(* Logix 5000 AddOnInstructionDefinition export BMC_AOI_PROC_BNI_XGx_x067_S5KV33_0325US; software revision 20.05 *)

TYPE BMC_UDT_BNI_XGx_x067_S5KV33_0325US :
STRUCT
   I : BMC_UDT_BNI_XGx_x067_IN_0325US;   // Master Input Data
   O : BMC_UDT_BNI_XGx_x067_OUT_0325US;   // Master Output Data
   C : BMC_UDT_BNI_XGx_x067_Config_0325US;   // Master Configuration Data
END_STRUCT
END_TYPE

TYPE BMC_UDT_BNI_XGx_x067_Dispaly_0325US :
STRUCT
   Red : BOOL;   // Set Display LEDs to Red
   Green : BOOL;   // Set Display LEDs to Green
   Lock : BOOL;   // Set Display Lock
END_STRUCT
END_TYPE

TYPE BMC_UDT_BNI_XGx_x067_OUT_0325US :
STRUCT
   DO : BMC_UDT_BNI_XGx_x067_Port_Pin_0325US;   // Master Digital Output
   Restart : BMC_UDT_BNI_XGx_x067_Port_Pin_0325US;   // Overload Restart
   Display : BMC_UDT_BNI_XGx_x067_Dispaly_0325US;   // Display LED and Display Lock
END_STRUCT
END_TYPE

TYPE BMC_UDT_BNI_XGx_x067_PortIOLDIag_0325US :
STRUCT
   X01 : BMC_UDT_BNI_XGx_x067_IOLDiagSub_0325US;   // IO-Link Diagnostics Port X01
   X02 : BMC_UDT_BNI_XGx_x067_IOLDiagSub_0325US;   // IO-Link Diagnostics Port X02
   X03 : BMC_UDT_BNI_XGx_x067_IOLDiagSub_0325US;   // IO-Link Diagnostics Port X03
   X04 : BMC_UDT_BNI_XGx_x067_IOLDiagSub_0325US;   // IO-Link Diagnostics Port X04
   X05 : BMC_UDT_BNI_XGx_x067_IOLDiagSub_0325US;   // IO-Link Diagnostics Port X05
   X06 : BMC_UDT_BNI_XGx_x067_IOLDiagSub_0325US;   // IO-Link Diagnostics Port X06
   X07 : BMC_UDT_BNI_XGx_x067_IOLDiagSub_0325US;   // IO-Link Diagnostics Port X07
   X08 : BMC_UDT_BNI_XGx_x067_IOLDiagSub_0325US;   // IO-Link Diagnostics Port X08
END_STRUCT
END_TYPE

TYPE BMC_UDT_BNI_XGx_x067_IOLDiagSub_0325US :
STRUCT
   Port_in_IOL_Mode : BOOL;   // Port in IO-Link Mode
   Device_Connected : BOOL;   // IO-Link Device Connected to Port
   Reserved_02 : BOOL;   // Reserved
   Reserved_03 : BOOL;   // Reserved
   Reserved_04 : BOOL;   // Reserved
   Reserved_05 : BOOL;   // Reserved
   Reserved_06 : BOOL;   // Reserved
   Reserved_07 : BOOL;   // Reserved
   Validation_Failed : BOOL;   // Validation Failed - Vendor or Device ID does not match conencted device
   DS_Validation_Failed : BOOL;   // Parameter Server Failed
   Process_Data_Invalid : BOOL;   // IO-Link Device Process Data Invalid
   Reserved_11 : BOOL;   // Reserved
   Reserved_12 : BOOL;   // Reserved
   Reserved_13 : BOOL;   // Reserved
   Reserved_14 : BOOL;   // Reserved
   IOL_Short_Circuit : BOOL;   // Short between Pin 4 and Pin 3 when in IO-Link Mode
   Vendor_ID_1 : SINT;   // Vendor ID
   Vendor_ID_2 : SINT;   // Vendor ID
   Device_ID_1 : SINT;   // Device ID
   Device_ID_2 : SINT;   // Device ID
   Device_ID_3 : SINT;   // Device ID
   Event_1_Mode_Type : SINT;   // Event Mode and Type
   Event_1_Code_High : SINT;   // Event Code High Byte
   Event_1_Code_Low : SINT;   // Event Code Low Byte
   Event_2_Mode_Type : SINT;   // Event Mode and Type
   Event_2_Code_High : SINT;   // Event Code High Byte
   Event_2_Code_Low : SINT;   // Event Code Low Byte
   Event_3_Mode_Type : SINT;   // Event Mode and Type
   Event_3_Code_High : SINT;   // Event Code High Byte
   Event_3_Code_Low : SINT;   // Event Code Low Byte
END_STRUCT
END_TYPE

TYPE BMC_UDT_BNI_XGx_x067_Config_0325US :
STRUCT
   Port_X01_Pin_4_Mode : BOOL;   // 0 - Disable IO-Link 1- Enable IO-Link
   Port_X01_Pin_2_Mode : BOOL;   // 0 - Pin 2 is switchable 1 - Pin 2 is ON Constant
   Port_X02_Pin_4_Mode : BOOL;   // 0 - Disable IO-Link 1- Enable IO-Link
   Port_X02_Pin_2_Mode : BOOL;   // 0 - Pin 2 is switchable 1 - Pin 2 is ON Constant
   Port_X03_Pin_4_Mode : BOOL;   // 0 - Disable IO-Link 1- Enable IO-Link
   Port_X03_Pin_2_Mode : BOOL;   // 0 - Pin 2 is switchable 1 - Pin 2 is ON Constant
   Port_X04_Pin_4_Mode : BOOL;   // 0 - Disable IO-Link 1- Enable IO-Link
   Port_X04_Pin_2_Mode : BOOL;   // 0 - Pin 2 is switchable 1 - Pin 2 is ON Constant
   Port_X05_Pin_4_Mode : BOOL;   // 0 - Disable IO-Link 1- Enable IO-Link
   Port_X05_Pin_2_Mode : BOOL;   // 0 - Pin 2 is switchable 1 - Pin 2 is ON Constant
   Port_X06_Pin_4_Mode : BOOL;   // 0 - Disable IO-Link 1- Enable IO-Link
   Port_X06_Pin_2_Mode : BOOL;   // 0 - Pin 2 is switchable 1 - Pin 2 is ON Constant
   Port_X07_Pin_4_Mode : BOOL;   // 0 - Disable IO-Link 1- Enable IO-Link
   Port_X07_Pin_2_Mode : BOOL;   // 0 - Pin 2 is switchable 1 - Pin 2 is ON Constant
   Port_X08_Pin_4_Mode : BOOL;   // 0 - Disable IO-Link 1- Enable IO-Link
   Port_X08_Pin_2_Mode : BOOL;   // 0 - Pin 2 is switchable 1 - Pin 2 is ON Constant
   Port_X01_Cycle_Time : SINT;   // Set Cycle Time (0 = Fastest Update Rate)
   Port_X01_Validation_Backup : SINT;   // 0 - No Validation or Parameter Server 1 - Validation Device 1.0 2 - Validation Device 1.1 3 - Parameter Server - Backup and Restore 4 - Parameter Server - Restore
   Port_X01_Vendor_ID_1 : SINT;   // Vendor ID High Byte - Used with Validation and Backup Parameter
   Port_X01_Vendor_ID_2 : SINT;   // Vendor ID Low Byte - Used with Validation and Backup Parameter
   Port_X01_Device_ID_1 : SINT;   // Device ID High Byte - Used with Validation and Backup Parameter
   Port_X01_Device_ID_2 : SINT;   // Device ID Middle Byte - Used with Validation and Backup Parameter
   Port_X01_Device_ID_3 : SINT;   // Device ID Low Byte - Used with Validation and Backup Parameter
   Port_X02_Cycle_Time : SINT;   // Set Cycle Time (0 = Fastest Update Rate)
   Port_X02_Validation_Backup : SINT;   // 0 - No Validation or Parameter Server 1 - Validation Device 1.0 2 - Validation Device 1.1 3 - Parameter Server - Backup and Restore 4 - Parameter Server - Restore
   Port_X02_Vendor_ID_1 : SINT;   // Vendor ID High Byte - Used with Validation and Backup Parameter
   Port_X02_Vendor_ID_2 : SINT;   // Vendor ID Low Byte - Used with Validation and Backup Parameter
   Port_X02_Device_ID_1 : SINT;   // Device ID High Byte - Used with Validation and Backup Parameter
   Port_X02_Device_ID_2 : SINT;   // Device ID Middle Byte - Used with Validation and Backup Parameter
   Port_X02_Device_ID_3 : SINT;   // Device ID Low Byte - Used with Validation and Backup Parameter
   Port_X03_Cycle_Time : SINT;   // Set Cycle Time (0 = Fastest Update Rate)
   Port_X03_Validation_Backup : SINT;   // 0 - No Validation or Parameter Server 1 - Validation Device 1.0 2 - Validation Device 1.1 3 - Parameter Server - Backup and Restore 4 - Parameter Server - Restore
   Port_X03_Vendor_ID_1 : SINT;   // Vendor ID High Byte - Used with Validation and Backup Parameter
   Port_X03_Vendor_ID_2 : SINT;   // Vendor ID Low Byte - Used with Validation and Backup Parameter
   Port_X03_Device_ID_1 : SINT;   // Device ID High Byte - Used with Validation and Backup Parameter
   Port_X03_Device_ID_2 : SINT;   // Device ID Middle Byte - Used with Validation and Backup Parameter
   Port_X03_Device_ID_3 : SINT;   // Device ID Low Byte - Used with Validation and Backup Parameter
   Port_X04_Cycle_Time : SINT;   // Set Cycle Time (0 = Fastest Update Rate)
   Port_X04_Validation_Backup : SINT;   // 0 - No Validation or Parameter Server 1 - Validation Device 1.0 2 - Validation Device 1.1 3 - Parameter Server - Backup and Restore 4 - Parameter Server - Restore
   Port_X04_Vendor_ID_1 : SINT;   // Vendor ID High Byte - Used with Validation and Backup Parameter
   Port_X04_Vendor_ID_2 : SINT;   // Vendor ID Low Byte - Used with Validation and Backup Parameter
   Port_X04_Device_ID_1 : SINT;   // Device ID High Byte - Used with Validation and Backup Parameter
   Port_X04_Device_ID_2 : SINT;   // Device ID Middle Byte - Used with Validation and Backup Parameter
   Port_X04_Device_ID_3 : SINT;   // Device ID Low Byte - Used with Validation and Backup Parameter
   Port_X05_Cycle_Time : SINT;   // Set Cycle Time (0 = Fastest Update Rate)
   Port_X05_Validation_Backup : SINT;   // 0 - No Validation or Parameter Server 1 - Validation Device 1.0 2 - Validation Device 1.1 3 - Parameter Server - Backup and Restore 4 - Parameter Server - Restore
   Port_X05_Vendor_ID_1 : SINT;   // Vendor ID High Byte - Used with Validation and Backup Parameter
   Port_X05_Vendor_ID_2 : SINT;   // Vendor ID Low Byte - Used with Validation and Backup Parameter
   Port_X05_Device_ID_1 : SINT;   // Device ID High Byte - Used with Validation and Backup Parameter
   Port_X05_Device_ID_2 : SINT;   // Device ID Middle Byte - Used with Validation and Backup Parameter
   Port_X05_Device_ID_3 : SINT;   // Device ID Low Byte - Used with Validation and Backup Parameter
   Port_X06_Cycle_Time : SINT;   // Set Cycle Time (0 = Fastest Update Rate)
   Port_X06_Validation_Backup : SINT;   // 0 - No Validation or Parameter Server 1 - Validation Device 1.0 2 - Validation Device 1.1 3 - Parameter Server - Backup and Restore 4 - Parameter Server - Restore
   Port_X06_Vendor_ID_1 : SINT;   // Vendor ID High Byte - Used with Validation and Backup Parameter
   Port_X06_Vendor_ID_2 : SINT;   // Vendor ID Low Byte - Used with Validation and Backup Parameter
   Port_X06_Device_ID_1 : SINT;   // Device ID High Byte - Used with Validation and Backup Parameter
   Port_X06_Device_ID_2 : SINT;   // Device ID Middle Byte - Used with Validation and Backup Parameter
   Port_X06_Device_ID_3 : SINT;   // Device ID Low Byte - Used with Validation and Backup Parameter
   Port_X07_Cycle_Time : SINT;   // Set Cycle Time (0 = Fastest Update Rate)
   Port_X07_Validation_Backup : SINT;   // 0 - No Validation or Parameter Server 1 - Validation Device 1.0 2 - Validation Device 1.1 3 - Parameter Server - Backup and Restore 4 - Parameter Server - Restore
   Port_X07_Vendor_ID_1 : SINT;   // Vendor ID High Byte - Used with Validation and Backup Parameter
   Port_X07_Vendor_ID_2 : SINT;   // Vendor ID Low Byte - Used with Validation and Backup Parameter
   Port_X07_Device_ID_1 : SINT;   // Device ID High Byte - Used with Validation and Backup Parameter
   Port_X07_Device_ID_2 : SINT;   // Device ID Middle Byte - Used with Validation and Backup Parameter
   Port_X07_Device_ID_3 : SINT;   // Device ID Low Byte - Used with Validation and Backup Parameter
   Port_X08_Cycle_Time : SINT;   // Set Cycle Time (0 = Fastest Update Rate)
   Port_X08_Validation_Backup : SINT;   // 0 - No Validation or Parameter Server 1 - Validation Device 1.0 2 - Validation Device 1.1 3 - Parameter Server - Backup and Restore 4 - Parameter Server - Restore
   Port_X08_Vendor_ID_1 : SINT;   // Vendor ID High Byte - Used with Validation and Backup Parameter
   Port_X08_Vendor_ID_2 : SINT;   // Vendor ID Low Byte - Used with Validation and Backup Parameter
   Port_X08_Device_ID_1 : SINT;   // Device ID High Byte - Used with Validation and Backup Parameter
   Port_X08_Device_ID_2 : SINT;   // Device ID Middle Byte - Used with Validation and Backup Parameter
   Port_X08_Device_ID_3 : SINT;   // Device ID Low Byte - Used with Validation and Backup Parameter
END_STRUCT
END_TYPE

TYPE BMC_UDT_BNI_XGx_x067_Power_0325US :
STRUCT
   UA_Low : BOOL;   // UA Power Low (Less than 18 Volts)
   US_Low : BOOL;   // US Power Low (Less than 18 Volts)
   No_UA : BOOL;   // No UA Power (Less than 11 Volts)
END_STRUCT
END_TYPE

TYPE IO_Link_Port_Data :
STRUCT
   Inputs : SINT[48];
   Outputs : SINT[48];
END_STRUCT
END_TYPE

TYPE BMC_UDT_BNI_XGx_x067_Port_Pin_0325US :
STRUCT
   X01_00 : BOOL;   // Port X01 LED 00 (Pin 4)
   X01_01 : BOOL;   // Port X01 LED 01 (Pin 2)
   X02_00 : BOOL;   // Port X02 LED 00 (Pin 4)
   X02_01 : BOOL;   // Port X02 LED 01 (Pin 2)
   X03_00 : BOOL;   // Port X03 LED 00 (Pin 4)
   X03_01 : BOOL;   // Port X03 LED 01 (Pin 2)
   X04_00 : BOOL;   // Port X04 LED 00 (Pin 4)
   X04_01 : BOOL;   // Port X04 LED 01 (Pin 2)
   X05_00 : BOOL;   // Port X05 LED 00 (Pin 4)
   X05_01 : BOOL;   // Port X05 LED 01 (Pin 2)
   X06_00 : BOOL;   // Port X06 LED 00 (Pin 4)
   X06_01 : BOOL;   // Port X06 LED 01 (Pin 2)
   X07_00 : BOOL;   // Port X07 LED 00 (Pin 4)
   X07_01 : BOOL;   // Port X07 LED 01 (Pin 2)
   X08_00 : BOOL;   // Port X08 LED 00 (Pin 4)
   X08_01 : BOOL;   // Port X08 LED 01 (Pin 2)
END_STRUCT
END_TYPE

TYPE BMC_UDT_BNI_XGx_x067_IN_0325US :
STRUCT
   DI : BMC_UDT_BNI_XGx_x067_Port_Pin_0325US;   // Master Digital Inputs
   Short_Circuit : BMC_UDT_BNI_XGx_x067_Port_Pin_0325US;   // Master Short Circuit Diagnostic
   Overload : BMC_UDT_BNI_XGx_x067_Port_Pin_0325US;   // Master Overload Diagnostic
   Power_Fault : BMC_UDT_BNI_XGx_x067_Power_0325US;   // Master Power Diagnostic
   IOL_Diag : BMC_UDT_BNI_XGx_x067_PortIOLDIag_0325US;   // IO-Link Port Diagnostic
END_STRUCT
END_TYPE

ADD_ON_INSTRUCTION BMC_AOI_PROC_BNI_XGx_x067_S5KV33_0325US   (* revision 4.0 0325US, vendor Balluff Inc *)
// BNI XGx-5xx-xxx-x067 AOI for use with RSlogix version 18-20 and Studio 5K Version 34 and 35 if version 36 is not installed on user's PC.
// Revision note:
// -3.0 Release for testing
// -4.0 Initial Release
VAR_IN_OUT
   BNI_XGx_x067_Raw_Input_Data : SINT[392]; {required}
        [0].0   // Input Port 0 Pin 4
        [0].1   // Input Port 0 Pin 2
        [0].2   // Input Port 1 Pin 4
        [0].3   // Input Port 1 Pin 2
        [0].4   // Input Port 2 Pin 4
        [0].5   // Input Port 2 Pin 2
        [0].6   // Input Port 3 Pin 4
        [0].7   // Input Port 3 Pin 2
        [1].0   // Input Port 4 Pin 4
        [1].1   // Input Port 4 Pin 2
        [1].2   // Input Port 5 Pin 4
        [1].3   // Input Port 5 Pin 2
        [1].4   // Input Port 6 Pin 4
        [1].5   // Input Port 6 Pin 2
        [1].6   // Input Port 7 Pin 4
        [1].7   // Input Port 7 Pin 2
        [2].0   // Port 0 Pin 4 Short Circuit
        [2].1   // Port 0 Pin 2 Short Circuit
        [2].2   // Port 1 Pin 4 Short Circuit
        [2].3   // Port 1 Pin 2 Short Circuit
        [2].4   // Port 2 Pin 4 Short Circuit
        [2].5   // Port 2 Pin 2 Short Circuit
        [2].6   // Port 3 Pin 4 Short Circuit
        [2].7   // Port 3 Pin 2 Short Circuit
        [3].0   // Port 4 Pin 4 Short Circuit
        [3].1   // Port 4 Pin 2 Short Circuit
        [3].2   // Port 5 Pin 4 Short Circuit
        [3].3   // Port 5 Pin 2 Short Circuit
        [3].4   // Port 6 Pin 4 Short Circuit
        [3].5   // Port 6 Pin 2 Short Circuit
        [3].6   // Port 7 Pin 4 Short Circuit
        [3].7   // Port 7 Pin 2 Short Circuit
        [4].0   // Port 0 Pin 4 Output Overload Status
        [4].1   // Port 0 Pin 2 Output Overload Status
        [4].2   // Port 1 Pin 4 Output Overload Status
        [4].3   // Port 1 Pin 2 Output Overload Status
        [4].4   // Port 2 Pin 4 Output Overload Status
        [4].5   // Port 2 Pin 2 Output Overload Status
        [4].6   // Port 3 Pin 4 Output Overload Status
        [4].7   // Port 3 Pin 2 Output Overload Status
        [5].0   // Port 4 Pin 4 Output Overload Status
        [5].1   // Port 4 Pin 2 Output Overload Status
        [5].2   // Port 5 Pin 4 Output Overload Status
        [5].3   // Port 5 Pin 2 Output Overload Status
        [5].4   // Port 6 Pin 4 Output Overload Status
        [5].5   // Port 6 Pin 2 Output Overload Status
        [5].6   // Port 7 Pin 4 Output Overload Status
        [5].7   // Port 7 Pin 2 Output Overload Status
        [6].0   // Output Power from Aux Power cable Under Voltage
        [6].1   // Module Power from IO-Link Communication Cable Under Voltage
        [6].2   // Not used
        [6].3   // Not used
        [6].4   // Not used
        [6].5   // Not used
        [6].6   // Not used
        [6].7   // Not used
        [7]   // Port 1 Input Byte 0
        [8]   // Port 1 Input Byte 1
        [9]   // Port 1 Input Byte 2
        [10]   // Port 1 Input Byte 3
        [11]   // Port 1 Input Byte 4
        [32].0   // Port 1 EP bit Event Present
        [32].1   // Reserved
        [32].2   // Reserved
        [32].3   // Reserved
        [32].4   // Reserved
        [32].5   // Port 1 VF bit Validation Failed
        [32].6   // Port 1 DC bit Device Connected
        [32].7   // Port 1 IOL bit Port in IO-Link Mode
        [33].0   // Reserved
        [33].1   // Reserved
        [33].2   // Reserved
        [33].3   // Reserved
        [33].4   // Reserved
        [33].5   // Reserved
        [33].6   // Reserved
        [33].7   // Reserved
        [34]   // Port 1 Vendor ID Number Byte 1 (High byte)
        [35]   // Port 1 Vendor ID Number Byte 2 (Middle byte)
        [36]   // Port 1 Vendor ID Number Byte 3 (Low byte)
        [37]   // Port 1 Device ID Number Byte 1 (High byte)
        [38]   // Port 1 Device ID Number Byte 2 (Middle byte)
        [39]   // Port 1 Device ID Number Byte 3 (Low byte)
        [40].0   // Port 1 In I/O Link Mode
        [40].1   // Port 1 I/O Link Device Connected
        [41].0   // Port 1 I/O Link Device Configuration Mismatch
        [52]   // Port 1 Input Byte 46
        [53]   // Port 1 Input Byte 47
        [54]   // Port 1 Input Byte 48
        [55]   // Port 2 Input Byte 0
        [56]   // Port 2 Input Byte 1
        [57]   // Port 2 Input Byte 2
        [58]   // Port 2 Input Byte 3
        [59]   // Port 2 Input Byte 4
        [88].0   // Port 2 In I/O Link Mode
        [88].1   // Port 2 I/O Link Device Connected
        [89].0   // Port 2 I/O Link Device Configuration Mismatch
        [100]   // Port 2 Input Byte 46
        [101]   // Port 2 Input Byte 47
        [102]   // Port 2 Input Byte 48
        [103]   // Port 3 Input Byte 0
        [104]   // Port 3 Input Byte 1
        [105]   // Port 3 Input Byte 2
        [106]   // Port 3 Input Byte 3
        [107]   // Port 3 Input Byte 4
        [136].0   // Port 3 In I/O Link Mode
        [136].1   // Port 3 I/O Link Device Connected
        [137].0   // Port 3 I/O Link Device Configuration Mismatch
        [148]   // Port 3 Input Byte 46
        [149]   // Port 3 Input Byte 47
        [150]   // Port 3 Input Byte 48
        [151]   // Port 4 Input Byte 0
        [152]   // Port 4 Input Byte 1
        [153]   // Port 4 Input Byte 2
        [154]   // Port 4 Input Byte 3
        [184].0   // Port 4 In I/O Link Mode
        [184].1   // Port 4 I/O Link Device Connected
        [185].0   // Port 4 I/O Link Device Configuration Mismatch
        [196]   // Port 4 Input Byte 46
        [197]   // Port 4 Input Byte 47
        [198]   // Port 4 Input Byte 48
   BNI_XGx_x067_Raw_Output_Data : SINT[262]; {required}
        [0].0   // Output Port 0 Pin 4
        [0].1   // Output Port 0 Pin 2
        [0].2   // Output Port 1 Pin 4
        [0].3   // Output Port 1 Pin 2
        [0].4   // Output Port 2 Pin 4
        [0].5   // Output Port 2 Pin 2
        [0].6   // Output Port 3 Pin 4
        [0].7   // Output Port 3 Pin 2
        [1].0   // Output Port 4 Pin 4
        [1].1   // Output Port 4 Pin 2
        [1].2   // Output Port 5 Pin 4
        [1].3   // Output Port 5 Pin 2
        [1].4   // Output Port 6 Pin 4
        [1].5   // Output Port 6 Pin 2
        [1].6   // Output Port 7 Pin 4
        [1].7   // Output Port 7 Pin 2
        [2].0   // Port 0 Pin 4 Output Restart
        [2].1   // Port 0 Pin 2 Output Restart
        [2].2   // Port 1 Pin 4 Output Restart
        [2].3   // Port 1 Pin 2 Output Restart
        [2].4   // Port 2 Pin 4 Output Restart
        [2].5   // Port 2 Pin 2 Output Restart
        [2].6   // Port 3 Pin 4 Output Restart
        [2].7   // Port 3 Pin 2 Output Restart
        [3].0   // Port 4 Pin 4 Output Restart
        [3].1   // Port 4 Pin 2 Output Restart
        [3].2   // Port 5 Pin 4 Output Restart
        [3].3   // Port 5 Pin 2 Output Restart
        [3].4   // Port 6 Pin 4 Output Restart
        [3].5   // Port 6 Pin 2 Output Restart
        [3].6   // Port 7 Pin 4 Output Restart
        [3].7   // Port 7 Pin 2 Output Restart
        [4].0   // Red LED Display Output
        [4].1   // Green LED Display Output
        [4].2   // Lock Display Output
        [5]   // Port 1 Output Data Byte 0
        [6]   // Port 1 Output Data Byte 1
        [7]   // Port 1 Output Data Byte 2
        [8]   // Port 1 Output Data Byte 3
        [9]   // Port 1 Output Data Byte 4
        [10]   // Port 1 Output Data Byte 5
        [11]   // Port 1 Output Data Byte 6
        [12]   // Port 1 Output Data Byte 7
        [13]   // Port 1 Output Data Byte 8
        [14]   // Port 1 Output Data Byte 9
        [15]   // Port 1 Output Data Byte 10
        [16]   // Port 1 Output Data Byte 11
        [17]   // Port 1 Output Data Byte 12
        [18]   // Port 1 Output Data Byte 13
        [19]   // Port 1 Output Data Byte 14
        [20]   // Port 1 Output Data Byte 15
        [21]   // Port 1 Output Data Byte 16
        [22]   // Port 1 Output Data Byte 17
        [23]   // Port 1 Output Data Byte 18
        [24]   // Port 1 Output Data Byte 19
        [25]   // Port 1 Output Data Byte 20
        [26]   // Port 1 Output Data Byte 21
        [27]   // Port 1 Output Data Byte 22
        [28]   // Port 1 Output Data Byte 23
        [29]   // Port 1 Output Data Byte 24
        [30]   // Port 1 Output Data Byte 25
        [31]   // Port 1 Output Data Byte 26
        [32]   // Port 1 Output Data Byte 27
        [33]   // Port 1 Output Data Byte 28
        [34]   // Port 1 Output Data Byte 29
        [35]   // Port 1 Output Data Byte 30
        [36]   // Port 1 Output Data Byte 31
        [37]   // Port 2 Output Data Byte 0
        [38]   // Port 2 Output Data Byte 1
        [69]   // Port 3 Output Data Byte 0
        [70]   // Port 3 Output Data Byte 1
        [101]   // Port 4 Output Data Byte 0
        [102]   // Port 4 Output Data Byte 1
   BNI_XGx_x067_Raw_Config_Data : SINT[58]; {required}
        [1]   // Port 5 (Bits 0_1) Port 6 (Bits 2_3) Port 7 (Bits 4_5) Port 8 (Bits 6_7) Function Function 00d=0x00=Standrd I/O 01d=0x01=IO-Link Mod 02d=0x02=Fallback Md
        [2].0   // Parameter Data Conflict
        [2].1   // Enable Parameter Upload
        [2].2   // Enable Parameter Download
        [2].7   // Enable Parameter Server
        [3]   // RESERVED
        [4]   // Port 1 IO-Link Cycle Time Time (Bytes 5-0) Base (Bytes 7-6)
        [5]   // Port 1 Vendor ID Number Byte 1 High Byte
        [6]   // Port 1 Vendor ID Number Byte 2 Low Byte
        [7]   // Port 1 Device ID Number Byte 1 High Byte
        [8]   // Port 1 Device ID Number Byte 2 Middle Byte
        [9]   // Port 1 Device ID Number Byte 3 Low Byte
        [10]   // Port 2 IO-Link Cycle Time Time (Bytes 5-0) Base (Bytes 7-6)
        [11]   // Port 2 Vendor ID Number Byte 1 High Byte
        [12]   // Port 2 Vendor ID Number Byte 2 Low Byte
        [13]   // Port 2 Device ID Number Byte 1 High Byte
        [14]   // Port 2 Device ID Number Byte 2 Middle Byte
        [15]   // Port 2 Device ID Number Byte 3 Low Byte
        [16]   // Port 3 IO-Link Cycle Time Time (Bytes 5-0) Base (Bytes 7-6)
        [17]   // Port 3 Vendor ID Number Byte 1 High Byte
        [18]   // Port 3 Vendor ID Number Byte 2 Low Byte
        [19]   // Port 3 Device ID Number Byte 1 High Byte
        [20]   // Port 3 Device ID Number Byte 2 Middle Byte
        [21]   // Port 3 Device ID Number Byte 3 Low Byte
        [22]   // Port 4 IO-Link Cycle Time Time (Bytes 5-0) Base (Bytes 7-6)
        [23]   // Port 4 Vendor ID Number Byte 1 High Byte
        [24]   // Port 4 Vendor ID Number Byte 2 Low Byte
        [25]   // Port 1 Enable
        [25].1   // Port 1 Enable Upload Parameters
        [25].2   // Port 1 Enable Download Parameters
        [25].7   // Port 1 Enable Parameters Server
        [26]   // Port 4 Device ID Number Byte 2 Middle Byte
        [27]   // Port 4 Device ID Number Byte 3 Low Byte
        [49].1   // Port 2 Enable Upload Parameters
        [49].2   // Port 2 Enable Download Parameters
        [49].7   // Port 2 Enable Parameters Server
   BNI_XGx_x067_Port_X01_Data : IO_Link_Port_Data; {required}
        .INPUTS[0]   // Port X01 Input Data
   BNI_XGx_x067_Port_X02_Data : IO_Link_Port_Data; {required}
        .INPUTS[0]   // Port X02 Input Data
   BNI_XGx_x067_Port_X03_Data : IO_Link_Port_Data; {required}
        .INPUTS[0]   // Port X03 Input Data
   BNI_XGx_x067_Port_X04_Data : IO_Link_Port_Data; {required}
        .INPUTS[0]   // Port X04 Input Data
   BNI_XGx_x067_Port_X05_Data : IO_Link_Port_Data; {required}
   BNI_XGx_x067_Port_X06_Data : IO_Link_Port_Data; {required}
   BNI_XGx_x067_Port_X07_Data : IO_Link_Port_Data; {required}
   BNI_XGx_x067_Port_X08_Data : IO_Link_Port_Data; {required}
   Mapped_BNI_XGx_R067_Data : BMC_UDT_BNI_XGx_x067_S5KV33_0325US; {required}
END_VAR

ROUTINE Logic   (* ladder *)
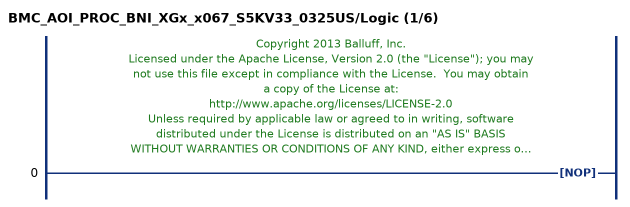
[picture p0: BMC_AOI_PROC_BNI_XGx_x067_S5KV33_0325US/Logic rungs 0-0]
   // Copyright 2013 Balluff, Inc.
   // Licensed under the Apache License, Version 2.0 (the "License"); you may
   // not use this file except in compliance with the License.  You may obtain
   // a copy of the License at:
   // http://www.apache.org/licenses/LICENSE-2.0
   // Unless required by applicable law or agreed to in writing, software
   // distributed under the License is distributed on an "AS IS" BASIS
   // WITHOUT WARRANTIES OR CONDITIONS OF ANY KIND, either express or
   // implied.  See the License for the specific language governing
   // permissions and limitations under the License.
   0: NOP();
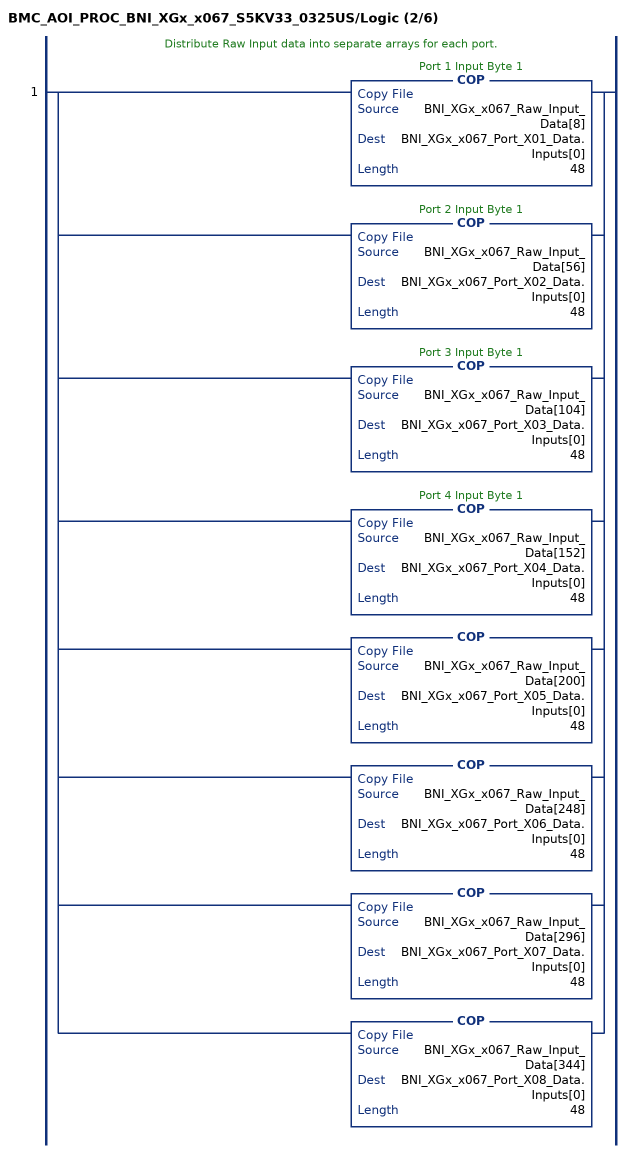
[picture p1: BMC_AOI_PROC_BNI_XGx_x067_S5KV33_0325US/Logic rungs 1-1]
   // Distribute Raw Input data into separate arrays for each port.
   1: [COP(BNI_XGx_x067_Raw_Input_Data[8],BNI_XGx_x067_Port_X01_Data.Inputs[0],48) ,COP(BNI_XGx_x067_Raw_Input_Data[56],BNI_XGx_x067_Port_X02_Data.Inputs[0],48) ,COP(BNI_XGx_x067_Raw_Input_Data[104],BNI_XGx_x067_Port_X03_Data.Inputs[0],48) ,COP(BNI_XGx_x067_Raw_Input_Data[152],BNI_XGx_x067_Port_X04_Data.Inputs[0],48) ,COP(BNI_XGx_x067_Raw_Input_Data[200],BNI_XGx_x067_Port_X05_Data.Inputs[0],48) ,COP(BNI_XGx_x067_Raw_Input_Data[248],BNI_XGx_x067_Port_X06_Data.Inputs[0],48) ,COP(BNI_XGx_x067_Raw_Input_Data[296],BNI_XGx_x067_Port_X07_Data.Inputs[0],48) ,COP(BNI_XGx_x067_Raw_Input_Data[344],BNI_XGx_x067_Port_X08_Data.Inputs[0],48) ];
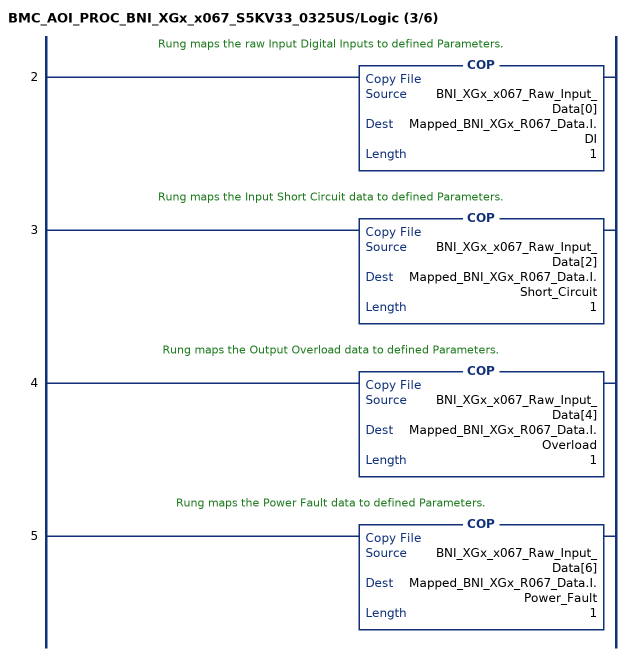
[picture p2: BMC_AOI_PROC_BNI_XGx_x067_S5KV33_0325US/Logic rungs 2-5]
   // Rung maps the raw Input Digital Inputs to defined Parameters.
   2: COP(BNI_XGx_x067_Raw_Input_Data[0],Mapped_BNI_XGx_R067_Data.I.DI,1);
   // Rung maps the Input Short Circuit data to defined Parameters.
   3: COP(BNI_XGx_x067_Raw_Input_Data[2],Mapped_BNI_XGx_R067_Data.I.Short_Circuit,1);
   // Rung maps the Output Overload data to defined Parameters.
   4: COP(BNI_XGx_x067_Raw_Input_Data[4],Mapped_BNI_XGx_R067_Data.I.Overload,1);
   // Rung maps the Power Fault data to defined Parameters.
   5: COP(BNI_XGx_x067_Raw_Input_Data[6],Mapped_BNI_XGx_R067_Data.I.Power_Fault,1);
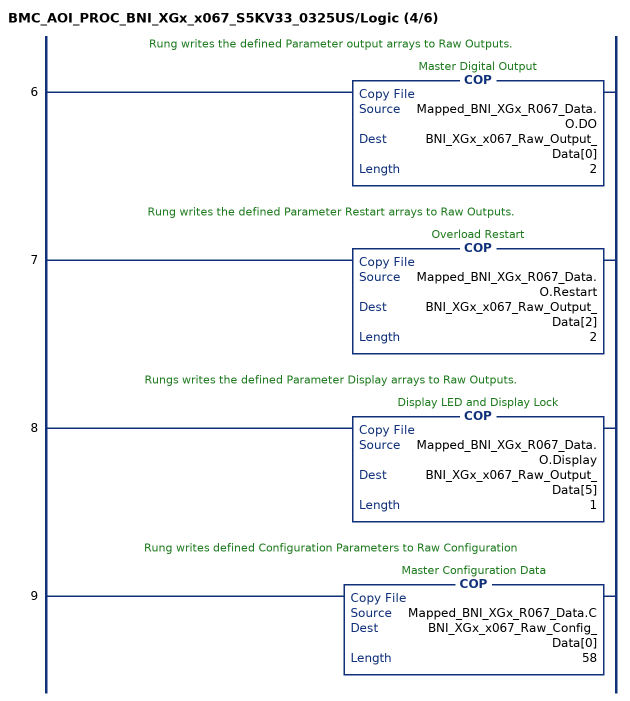
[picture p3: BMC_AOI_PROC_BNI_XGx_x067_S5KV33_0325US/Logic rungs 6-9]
   // Rung writes the defined Parameter output arrays to Raw Outputs.
   6: COP(Mapped_BNI_XGx_R067_Data.O.DO,BNI_XGx_x067_Raw_Output_Data[0],2);
   // Rung writes the defined Parameter Restart arrays to Raw Outputs.
   7: COP(Mapped_BNI_XGx_R067_Data.O.Restart,BNI_XGx_x067_Raw_Output_Data[2],2);
   // Rungs writes the defined Parameter Display arrays to Raw Outputs.
   8: COP(Mapped_BNI_XGx_R067_Data.O.Display,BNI_XGx_x067_Raw_Output_Data[5],1);
   // Rung writes defined Configuration Parameters to Raw Configuration
   9: COP(Mapped_BNI_XGx_R067_Data.C,BNI_XGx_x067_Raw_Config_Data[0],58);
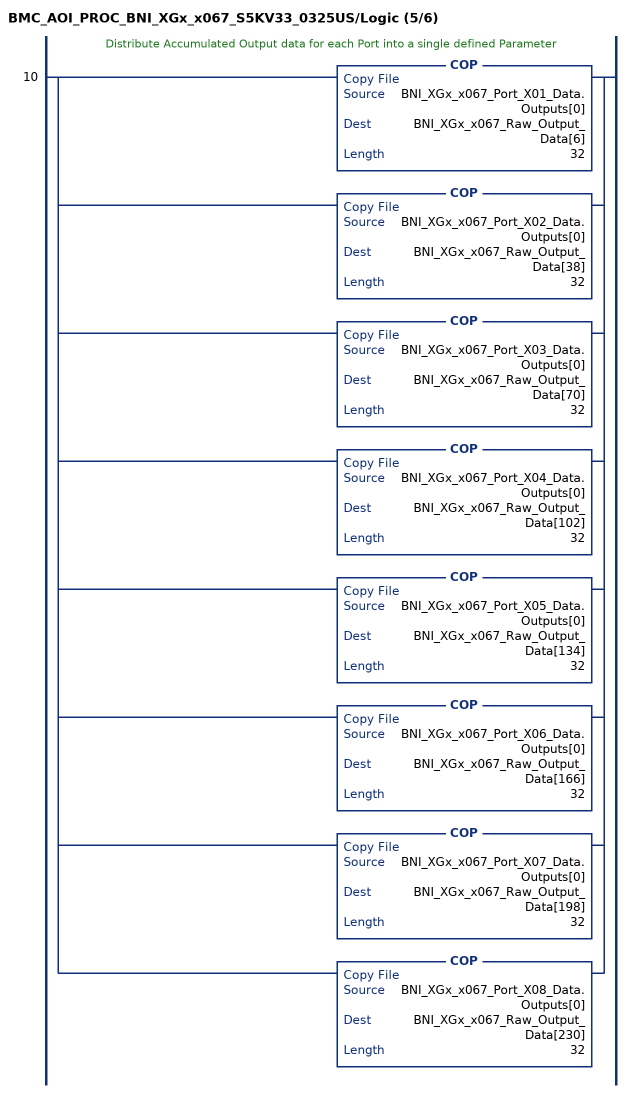
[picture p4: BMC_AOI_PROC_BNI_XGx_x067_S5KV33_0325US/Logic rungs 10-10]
   // Distribute Accumulated Output data for each Port into a single defined Parameter
   10: [COP(BNI_XGx_x067_Port_X01_Data.Outputs[0],BNI_XGx_x067_Raw_Output_Data[6],32) ,COP(BNI_XGx_x067_Port_X02_Data.Outputs[0],BNI_XGx_x067_Raw_Output_Data[38],32) ,COP(BNI_XGx_x067_Port_X03_Data.Outputs[0],BNI_XGx_x067_Raw_Output_Data[70],32) ,COP(BNI_XGx_x067_Port_X04_Data.Outputs[0],BNI_XGx_x067_Raw_Output_Data[102],32) ,COP(BNI_XGx_x067_Port_X05_Data.Outputs[0],BNI_XGx_x067_Raw_Output_Data[134],32) ,COP(BNI_XGx_x067_Port_X06_Data.Outputs[0],BNI_XGx_x067_Raw_Output_Data[166],32) ,COP(BNI_XGx_x067_Port_X07_Data.Outputs[0],BNI_XGx_x067_Raw_Output_Data[198],32) ,COP(BNI_XGx_x067_Port_X08_Data.Outputs[0],BNI_XGx_x067_Raw_Output_Data[230],32) ];
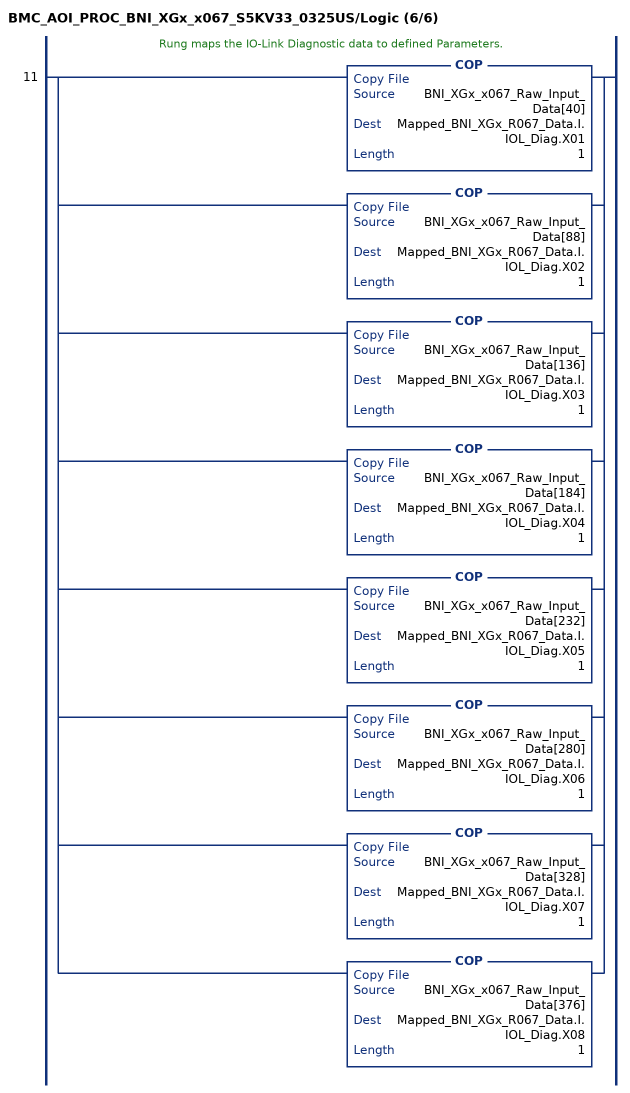
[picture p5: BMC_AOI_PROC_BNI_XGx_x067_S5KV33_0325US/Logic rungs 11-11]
   // Rung maps the IO-Link Diagnostic data to defined Parameters.
   11: [COP(BNI_XGx_x067_Raw_Input_Data[40],Mapped_BNI_XGx_R067_Data.I.IOL_Diag.X01,1) ,COP(BNI_XGx_x067_Raw_Input_Data[88],Mapped_BNI_XGx_R067_Data.I.IOL_Diag.X02,1) ,COP(BNI_XGx_x067_Raw_Input_Data[136],Mapped_BNI_XGx_R067_Data.I.IOL_Diag.X03,1) ,COP(BNI_XGx_x067_Raw_Input_Data[184],Mapped_BNI_XGx_R067_Data.I.IOL_Diag.X04,1) ,COP(BNI_XGx_x067_Raw_Input_Data[232],Mapped_BNI_XGx_R067_Data.I.IOL_Diag.X05,1) ,COP(BNI_XGx_x067_Raw_Input_Data[280],Mapped_BNI_XGx_R067_Data.I.IOL_Diag.X06,1) ,COP(BNI_XGx_x067_Raw_Input_Data[328],Mapped_BNI_XGx_R067_Data.I.IOL_Diag.X07,1) ,COP(BNI_XGx_x067_Raw_Input_Data[376],Mapped_BNI_XGx_R067_Data.I.IOL_Diag.X08,1) ];
END_ROUTINE
END_ADD_ON_INSTRUCTION
